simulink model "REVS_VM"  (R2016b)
settings: Solver=ode3  StartTime=REVS.sim_start_time_secs  StopTime=Inf  FixedStep=REVS.sim_step_time_secs  MaxStep=REVS.sim_step_time_secs  EnableMultiTasking=on
StopFcn:
  | postproc_datalog;
  | postproc_audit;
  | postproc_result;
model workspace (MATLAB code in the model file):
  other statements: REVS_setup_variants
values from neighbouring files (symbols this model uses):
  accessory = class_accessory_data    [class_test_data.m]
  battery = class_battery_data    [class_accessory_data.m]    (also in class_REVS_electric.m = class_REVS_battery)
  brake = struct(	'max_torque_Nm',[], 						'proportion_norm',1.0, 						'inertia_kgm2',0.0)    [class_REVS_drive_axle.m]
  engine = class_engine_data    [class_test_data.m]
  final_drive = struct(	'gear_ratio',[], 								'efficiency_norm',[], 								'inertia_kgm2',[] )    [class_REVS_drive_axle.m]
  gear = class_REVS_gearbox    [class_REVS_AT_transmission.m]
  tire = struct(	'radius_m',[], 						'rolling_resistance_coefficient',0, 						'vehicle_weight_norm',1.0,  						'wheel_slip_torque_Nm',[],  						'inertia_kgm2',0.0)    [class_REVS_drive_axle.m]
  torque_converter = class_REVS_torque_converter    [class_REVS_AT_transmission.m]
  transmission = class_transmission_data    [class_test_data.m]
  vehicle = class_vehicle_data    [class_test_data.m]
undefined symbols (not defined in the file or in its folder): alternator, ambient, controls, convert, DelayTimeSecs, drive_cycle, driver, electric, gear_strategy, InitialCondition, InitialValue, LoadSource, LookupStructure, MultiplyPosInputs, Normalize, NumPhases, REVS, SpeedSource, starter, tableshift, UpperSaturationLimit, Value, VerboseLevel, VerboseSignal
libraries: simulink x153
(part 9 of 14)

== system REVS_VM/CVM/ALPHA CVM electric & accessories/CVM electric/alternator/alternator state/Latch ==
  On : Inport  PortDimensions=1
  Off : Inport  Port=2  PortDimensions=1
  Combinatorial  Logic : CombinatorialLogic  TruthTable=[0;1;0;0;1;1;(tb==2);(tb>=2)]
  Memory2 : Memory  X0=InitialCondition
  Mux : Mux  Inputs=3
  State : Outport  PortDimensions=1
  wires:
  Off/1 -> Mux/2
  On/1 -> Mux/1
  Memory2/1 -> Mux/3
  Mux/1 -> Combinatorial  Logic/1
  Combinatorial  Logic/1 -> State/1, Memory2/1

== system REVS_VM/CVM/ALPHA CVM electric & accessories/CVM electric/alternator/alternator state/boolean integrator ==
  bool : Inport
  Constant : Constant  Value=Normalize
  Data Type Conversion2 : DataTypeConversion  OutDataTypeStr=double
  Integrator1 : Integrator  ExternalReset=falling  LimitOutput=on  UpperSaturationLimit=UpperSaturationLimit  LowerSaturationLimit=0
  Switch : Switch  Criteria=u2 > Threshold
  normalize : Gain  Gain=1/UpperSaturationLimit
  out : Outport
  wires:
  Switch/1 -> out/1
  normalize/1 -> Switch/1
  Integrator1/1 -> Switch/3, normalize/1
  Constant/1 -> Switch/2
  bool/1 -> Data Type Conversion2/1
  Data Type Conversion2/1 -> Integrator1/1, Integrator1/2

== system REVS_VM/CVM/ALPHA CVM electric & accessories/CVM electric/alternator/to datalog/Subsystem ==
  In1 : Inport
  Enable : EnablePort
  To Workspace : ToWorkspace  VariableName=datalog__alternator__regen_SOC_state  SampleTime=-1
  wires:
  In1/1 -> To Workspace/1

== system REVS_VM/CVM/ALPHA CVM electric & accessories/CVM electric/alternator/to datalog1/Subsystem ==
  In1 : Inport
  Enable : EnablePort
  To Workspace : ToWorkspace  VariableName=datalog__alternator__target_voltage  SampleTime=-1
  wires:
  In1/1 -> To Workspace/1

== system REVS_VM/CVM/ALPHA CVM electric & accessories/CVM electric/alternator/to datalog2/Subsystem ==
  In1 : Inport
  Enable : EnablePort
  To Workspace : ToWorkspace  VariableName=datalog__alternator__state  SampleTime=-1
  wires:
  In1/1 -> To Workspace/1

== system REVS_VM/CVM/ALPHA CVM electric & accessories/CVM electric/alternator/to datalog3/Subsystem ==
  In1 : Inport
  Enable : EnablePort
  To Workspace : ToWorkspace  VariableName=datalog__alternator__regen_state  SampleTime=-1
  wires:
  In1/1 -> To Workspace/1

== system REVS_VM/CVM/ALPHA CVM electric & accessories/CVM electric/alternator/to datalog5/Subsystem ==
  In1 : Inport
  Enable : EnablePort
  To Workspace : ToWorkspace  VariableName=datalog__alternator__upshift_sig  SampleTime=-1
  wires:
  In1/1 -> To Workspace/1

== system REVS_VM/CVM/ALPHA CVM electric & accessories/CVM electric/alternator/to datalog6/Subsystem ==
  In1 : Inport
  Enable : EnablePort
  To Workspace : ToWorkspace  VariableName=datalog__alternator__voltage_boost  SampleTime=-1
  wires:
  In1/1 -> To Workspace/1

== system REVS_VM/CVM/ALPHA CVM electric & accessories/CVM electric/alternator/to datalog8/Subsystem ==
  In1 : Inport
  Enable : EnablePort
  To Workspace : ToWorkspace  VariableName=datalog__alternator__PID_current_A  SampleTime=-1
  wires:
  In1/1 -> To Workspace/1

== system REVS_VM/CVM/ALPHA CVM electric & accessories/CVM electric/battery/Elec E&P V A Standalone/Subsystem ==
  volts_V : Inport
  curr_A : Inport  Port=2
  Enable : EnablePort  ZeroCross=off
  Elec Energy V A : Subsystem  TreatAsAtomicUnit=on
  amps_to_workspace : ToWorkspace  VariableName=audit__elec__battery_Amps  SampleTime=-1
  energy_to_workspace : ToWorkspace  VariableName=audit__elec__battery_kJ  SampleTime=-1
  neg_energy_to_workspace : ToWorkspace  VariableName=audit__elec__battery_neg_kJ  SampleTime=-1
  pos_energy_to_workspace : ToWorkspace  VariableName=audit__elec__battery_pos_kJ  SampleTime=-1
  power_to_workspace : ToWorkspace  VariableName=audit__elec__battery_kW  SampleTime=-1
  volts_to_workspace : ToWorkspace  VariableName=audit__elec__battery_Volts  SampleTime=-1
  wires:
  Elec Energy V A/1("total_kJ ") -> energy_to_workspace/1
  Elec Energy V A/4(pwr_kW) -> power_to_workspace/1
  Elec Energy V A/2("pos_kJ ") -> pos_energy_to_workspace/1
  Elec Energy V A/3(neg_kJ) -> neg_energy_to_workspace/1
  curr_A/1 -> amps_to_workspace/1, Elec Energy V A/2(curr_A)
  volts_V/1 -> volts_to_workspace/1, Elec Energy V A/1(volts_V)

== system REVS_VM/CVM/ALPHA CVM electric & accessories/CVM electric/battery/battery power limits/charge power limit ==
  bus : Inport
  Bus Selector : BusSelector  OutputSignals=gb.gb_cmd_gear,gb_spd_in_radps,ctrl.gb_line_press_bar
  Lookup : Lookup_n-D  NumberOfTableDimensions=10  BreakpointsForDimension1=LookupStructure.axis_1.breakpoints  BreakpointsForDimension2=LookupStructure.axis_2.breakpoints  BreakpointsForDimension3=LookupStructure.axis_3.breakpoints  BreakpointsForDimension4=LookupStructure.axis_4.breakpoints  BreakpointsForDimension5=LookupStructure.axis_5.breakpoints  BreakpointsForDimension6=LookupStructure.axis_6.breakpoints  BreakpointsForDimension7=LookupStructure.axis_7.breakpoints  BreakpointsForDimension8=LookupStructure.axis_8.breakpoints  BreakpointsForDimension9=LookupStructure.axis_9.breakpoints  BreakpointsForDimension10=LookupStructure.axis_10.breakpoints  IndexSearchMethod=Linear search  BeginIndexSearchUsingPreviousIndexResult=on  Table=LookupStructure.table  InternalRulePriority=Speed  RndMeth=Simplest  SupportTunableTableSize=on  MaximumIndicesForEachDimension=LookupStructure.table_size
  out : Outport
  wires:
  bus/1 -> Bus Selector/1
  Lookup/1 -> out/1

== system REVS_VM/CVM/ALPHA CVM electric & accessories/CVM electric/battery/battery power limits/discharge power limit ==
  bus : Inport
  Bus Selector : BusSelector  OutputSignals=gb.gb_cmd_gear,gb_spd_in_radps,ctrl.gb_line_press_bar
  Lookup : Lookup_n-D  NumberOfTableDimensions=10  BreakpointsForDimension1=LookupStructure.axis_1.breakpoints  BreakpointsForDimension2=LookupStructure.axis_2.breakpoints  BreakpointsForDimension3=LookupStructure.axis_3.breakpoints  BreakpointsForDimension4=LookupStructure.axis_4.breakpoints  BreakpointsForDimension5=LookupStructure.axis_5.breakpoints  BreakpointsForDimension6=LookupStructure.axis_6.breakpoints  BreakpointsForDimension7=LookupStructure.axis_7.breakpoints  BreakpointsForDimension8=LookupStructure.axis_8.breakpoints  BreakpointsForDimension9=LookupStructure.axis_9.breakpoints  BreakpointsForDimension10=LookupStructure.axis_10.breakpoints  IndexSearchMethod=Linear search  BeginIndexSearchUsingPreviousIndexResult=on  Table=LookupStructure.table  InternalRulePriority=Speed  RndMeth=Simplest  SupportTunableTableSize=on  MaximumIndicesForEachDimension=LookupStructure.table_size
  out : Outport
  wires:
  bus/1 -> Bus Selector/1
  Lookup/1 -> out/1

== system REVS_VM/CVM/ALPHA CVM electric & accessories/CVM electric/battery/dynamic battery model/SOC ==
  batt_curr_A : Inport
  batt_temp_degC : Inport  Port=2
  Bus Creator : BusCreator  Inputs=2
  Divide1 : Product  Inputs=*/
  Integrator : Integrator  InitialConditionSource=external  InitialCondition=battery.initial_soc_norm * battery.capacity_Coulombs  LimitOutput=on  UpperSaturationLimit=battery.capacity_Coulombs  LowerSaturationLimit=0
  Negative Gain1 : Gain  Gain=-1
  Product : Product
  Product1 : Product
  Switch : Switch  OutDataTypeStr=double
  capacity (Coulombs) : Constant  Value=battery.capacity_Coulombs
  charge efficiency dynamic : Subsystem
  initial SoC : Constant  Value=battery.initial_soc_norm
  to datalog with base name : Subsystem
  SoC_norm : Outport
  chg_eff_norm : Outport  Port=2
  pile_curr_A : Outport  Port=3
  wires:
  initial SoC/1 -> Product1/1
  Product1/1 -> Integrator/2
  Divide1/1 -> to datalog with base name/1(Var), Bus Creator/2, SoC_norm/1  "soc_norm"
  capacity (Coulombs)/1 -> Divide1/2, Product1/2
  Integrator/1 -> Divide1/1
  batt_temp_degC/1 -> Bus Creator/1  "temp_degC"
  batt_curr_A/1 -> Product/1, Switch/1, Switch/2
  Switch/1 -> Negative Gain1/1
  Product/1 -> Switch/3
  Negative Gain1/1 -> pile_curr_A/1, Integrator/1
  charge efficiency dynamic/1(out) -> chg_eff_norm/1, Product/2
  Bus Creator/1 -> charge efficiency dynamic/1(bus)

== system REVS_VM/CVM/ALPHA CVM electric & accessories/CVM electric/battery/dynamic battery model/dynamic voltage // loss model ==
  batt_curr_A : Inport
  SoC_norm : Inport  Port=2
  batt_temp_degC : Inport  Port=3
  chg_eff_norm : Inport  Port=4
  pile_curr_A : Inport  Port=5
  Add1 : Sum
  Add2 : Sum  Inputs=+-
  Bus Creator : BusCreator  Inputs=4
  Divide : Product  Inputs=*/
  Gain3 : Gain  Gain=battery.voltage_transient_cal_norm
  Gain4 : Gain  Gain=1/1000
  Gain5 : Gain  Gain=1/1000
  Integrator1 : Integrator  ZeroCross=off
  Integrator2 : Integrator  ZeroCross=off
  Integrator3 : Integrator  ZeroCross=off
  Product : Product
  Product1 : Product
  RC long term (LT) : Subsystem
  RC short term (ST) : Subsystem
  Rs : Subsystem
  Subtract1 : Sum  Inputs=+++
  battery energy change : Subsystem
  battery energy discharge gross : Subsystem
  battery loss : Subsystem
  battery loss1 : Subsystem
  charge loss : Subsystem
  model : Subsystem
  negative : Saturate  UpperLimit=0  LowerLimit=-Inf
  num parallels : Constant  Value=battery.num_parallel_cells
  open circuit (pile) voltage : Subsystem
  result integrator : Subsystem
  OCV_V : Outport
  batt_volts_V : Outport  Port=2
  dis_res_Ohm : Outport  Port=3
  chg_res_Ohm : Outport  Port=4
  loss_pwr_W : Outport  Port=5
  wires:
  Gain5/1 -> Integrator1/1, result integrator/1(in), negative/1
  negative/1 -> Integrator3/1
  Integrator3/1 -> battery energy discharge gross/1(Var)
  chg_eff_norm/1 -> charge loss/1(charge_eff_norm)
  Add1/1 -> loss_pwr_W/1, Integrator2/1
  Add2/1 -> Gain3/1
  RC long term (LT)/1(RC_LT_V) -> Subtract1/2
  batt_temp_degC/1 -> Bus Creator/3  "temp_degC"
  RC short term (ST)/1(RC_ST_V) -> Subtract1/1
  Rs/1(Rs_V) -> Subtract1/3
  SoC_norm/1 -> Bus Creator/1  "soc_norm"
  Rs/2(Rs_dis_Ohm) -> dis_res_Ohm/1
  Rs/3(Rs_chg_Ohm) -> chg_res_Ohm/1
  pile_curr_A/1 -> Product/2
  Product/1 -> Gain5/1
  Integrator1/1 -> battery energy change/1(Var)
  Subtract1/1 -> Add2/2, Product1/2
  open circuit (pile) voltage/1(OCV_V) -> battery loss1/1(Var), Product/1, charge loss/3(OCV_V), Add2/1, OCV_V/1
  Divide/1 -> Bus Creator/2  "cell_curr_A"
  num parallels/1 -> Divide/2
  batt_curr_A/1 -> Bus Creator/4, charge loss/2(pack_curr_A), Divide/1, Product1/1  "pack_curr_A"
  Integrator2/1 -> Gain4/1
  charge loss/1(chg_loss_pwr_W) -> Add1/2
  Product1/1 -> Add1/1
  Gain4/1 -> battery loss/1(Var)
  Bus Creator/1 -> Rs/1(bus_in), RC long term (LT)/1(bus_in), RC short term (ST)/1(bus_in), open circuit (pile) voltage/1(bus_in)
  Gain3/1 -> batt_volts_V/1

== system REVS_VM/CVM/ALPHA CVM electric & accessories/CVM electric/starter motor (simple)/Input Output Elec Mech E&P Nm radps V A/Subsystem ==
  volts_in_V : Inport
  curr_in_A : Inport  Port=2
  trq_out_Nm : Inport  Port=3
  spd_out_radps : Inport  Port=4
  iner_out_kgm2 : Inport  Port=5
  Enable : EnablePort
  Elec E&P V A : Subsystem
  Loss_KJ_to_workspace : ToWorkspace  VariableName=audit__mech__starter__loss_kJ  SampleTime=-1
  Mech E&P Nm radps : Subsystem
  Pos : Saturate  UpperLimit=Inf  LowerLimit=0  ZeroCross=off
  Pos2 : Saturate  UpperLimit=Inf  LowerLimit=0  ZeroCross=off
  Sum : Sum  Inputs=+-|
  Sum1 : Sum  Inputs=|-+
  Sum2 : Sum
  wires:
  Pos2/1 -> Sum2/1
  Pos/1 -> Sum2/2
  trq_out_Nm/1 -> Mech E&P Nm radps/1(" trq_Nm")
  spd_out_radps/1 -> Mech E&P Nm radps/2(spd_radps)
  volts_in_V/1 -> Elec E&P V A/1(volts_V)
  curr_in_A/1 -> Elec E&P V A/2(curr_A)
  iner_out_kgm2/1 -> Mech E&P Nm radps/3(iner_kgm2)
  Mech E&P Nm radps/1(pos_kJ) -> Sum/2
  Elec E&P V A/2(neg_kJ) -> Sum1/1
  Mech E&P Nm radps/2(neg_kJ) -> Sum1/2
  Sum/1 -> Pos/1
  Sum1/1 -> Pos2/1
  Sum2/1 -> Loss_KJ_to_workspace/1
  Elec E&P V A/1(pos_kJ) -> Sum/1

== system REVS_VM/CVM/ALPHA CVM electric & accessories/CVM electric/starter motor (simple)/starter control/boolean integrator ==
  bool : Inport
  Constant : Constant  Value=Normalize
  Data Type Conversion2 : DataTypeConversion  OutDataTypeStr=double
  Integrator1 : Integrator  ExternalReset=falling  LimitOutput=on  UpperSaturationLimit=UpperSaturationLimit  LowerSaturationLimit=0
  Switch : Switch  Criteria=u2 > Threshold
  normalize : Gain  Gain=1/UpperSaturationLimit
  out : Outport
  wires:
  Switch/1 -> out/1
  normalize/1 -> Switch/1
  Integrator1/1 -> Switch/3, normalize/1
  Constant/1 -> Switch/2
  bool/1 -> Data Type Conversion2/1
  Data Type Conversion2/1 -> Integrator1/1, Integrator1/2

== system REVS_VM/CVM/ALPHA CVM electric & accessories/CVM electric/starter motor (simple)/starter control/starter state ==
  On : Inport  PortDimensions=1
  Off : Inport  Port=2  PortDimensions=1
  Combinatorial  Logic : CombinatorialLogic  TruthTable=[0;1;0;0;1;1;(tb==2);(tb>=2)]
  Memory2 : Memory  X0=InitialCondition
  Mux : Mux  Inputs=3
  State : Outport  PortDimensions=1
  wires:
  Off/1 -> Mux/2
  On/1 -> Mux/1
  Memory2/1 -> Mux/3
  Mux/1 -> Combinatorial  Logic/1
  Combinatorial  Logic/1 -> State/1, Memory2/1

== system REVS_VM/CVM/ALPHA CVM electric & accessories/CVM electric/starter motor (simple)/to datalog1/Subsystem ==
  In1 : Inport
  Enable : EnablePort
  To Workspace : ToWorkspace  VariableName=datalog__electric__starter_PID_torque_Nm  SampleTime=-1
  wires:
  In1/1 -> To Workspace/1

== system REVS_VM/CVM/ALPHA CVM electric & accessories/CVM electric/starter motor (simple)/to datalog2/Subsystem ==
  In1 : Inport
  Enable : EnablePort
  To Workspace : ToWorkspace  VariableName=datalog__electric__starter_state  SampleTime=-1
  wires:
  In1/1 -> To Workspace/1

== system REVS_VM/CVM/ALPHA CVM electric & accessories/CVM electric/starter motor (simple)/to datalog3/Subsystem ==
  In1 : Inport
  Enable : EnablePort
  To Workspace : ToWorkspace  VariableName=datalog__electric__starter_desired_torque_Nm  SampleTime=-1
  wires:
  In1/1 -> To Workspace/1

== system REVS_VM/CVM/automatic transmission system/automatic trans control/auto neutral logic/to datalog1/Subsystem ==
  In1 : Inport
  Enable : EnablePort
  To Workspace : ToWorkspace  VariableName=datalog__transmission__auto_neutral_command_bool  SampleTime=-1
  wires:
  In1/1 -> To Workspace/1

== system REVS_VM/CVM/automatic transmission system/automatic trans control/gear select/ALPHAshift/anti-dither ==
  raw : Inport
  Abs : Abs
  Memory : Memory
  Rounding Function : Rounding  Operator=round
  Sum : Sum  Inputs=|+-
  Switch : Switch  Criteria=u2 > Threshold  Threshold=.66
  low pass filter : TransferFcn  Denominator=[0.02 1]
  to datalog17 : Subsystem
  to datalog18 : Subsystem
  out : Outport
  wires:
  raw/1 -> to datalog18/1(Var), low pass filter/1
  low pass filter/1 -> Rounding Function/1, Sum/1, to datalog17/1(Var)
  Rounding Function/1 -> Switch/1
  Switch/1 -> out/1, Memory/1
  Sum/1 -> Abs/1
  Memory/1 -> Sum/2, Switch/3
  Abs/1 -> Switch/2

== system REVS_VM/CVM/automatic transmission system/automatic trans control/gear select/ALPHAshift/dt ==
  Clock : Clock
  Memory1 : Memory
  Sum : Sum  Inputs=|-+
  dt : Outport
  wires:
  Clock/1 -> Sum/2, Memory1/1
  Memory1/1 -> Sum/1
  Sum/1 -> dt/1

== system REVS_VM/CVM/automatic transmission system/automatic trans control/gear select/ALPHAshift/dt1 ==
  Clock : Clock
  Memory1 : Memory
  Sum : Sum  Inputs=|-+
  dt : Outport
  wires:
  Clock/1 -> Sum/2, Memory1/1
  Memory1/1 -> Sum/1
  Sum/1 -> dt/1

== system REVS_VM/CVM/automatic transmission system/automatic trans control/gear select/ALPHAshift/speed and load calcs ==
  eng_load_Nm : Inport
  trans_spd_in_radps : Inport  Port=2
  trans_spd_out_radps : Inport  Port=3
  eng_spd_radps : Inport  Port=4
  trans_gear_ratios : Inport  Port=5
  Logical Operator : Logic  Operator=NOT  AllPortsSameDT=off  OutDataTypeStr=boolean
  MinMax : MinMax  Inputs=2  ZeroCross=off
  MinMax1 : MinMax  Function=max  ZeroCross=off
  MinMax2 : MinMax  Function=max  Inputs=2  ZeroCross=off
  Product1 : Product  Inputs=***/
  Product2 : Product  Inputs=***
  Product3 : Product  Inputs=*/
  Product4 : Product  Inputs=***/
  Product5 : Product  Inputs=**
  Sum : Sum  Inputs=|++
  cost map : Lookup_n-D  BreakpointsForDimension1=gear_strategy.cost_map_torque_Nm  BreakpointsForDimension2=gear_strategy.cost_map_speed_radps  IndexSearchMethod=Linear search  BeginIndexSearchUsingPreviousIndexResult=on  Table=gear_strategy.cost_map  ExtrapMethod=Clip  UseLastTableValue=on  RndMeth=Simplest
  eps1 : Saturate  UpperLimit=Inf  LowerLimit=eps
  eps2 : Saturate  UpperLimit=Inf  LowerLimit=eps  ZeroCross=off
  eps3 : Saturate  UpperLimit=Inf  LowerLimit=eps
  max input torque : Lookup_n-D  NumberOfTableDimensions=1  BreakpointsForDimension1=gear_strategy.max_input_torque_speeds_radps  IndexSearchMethod=Linear search  BeginIndexSearchUsingPreviousIndexResult=on  Table=gear_strategy.max_input_torque_curve_Nm  ExtrapMethod=Clip  UseLastTableValue=on  RndMeth=Simplest
  non-neutral gears vector : simulink/Logic and Bit Operations/Compare To Zero  relop=~=  OutDataTypeStr=boolean
  non-neutral gears vector1 : simulink/Logic and Bit Operations/Compare To Zero  relop=~=  OutDataTypeStr=boolean
  speed mask : Constant  Value=gear_strategy.use_engine_speed_mask
  gear_trq_Nm : Outport
  gear_spd_radps : Outport  Port=2
  gear_cost : Outport  Port=3
  gear_avail_trq_Nm : Outport  Port=4
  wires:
  Product4/1 -> Sum/2  "engine_speeds"
  Product2/1 -> Sum/1  "speeds"
  eps3/1 -> Product4/4
  eng_spd_radps/1 -> Product1/3, MinMax2/2
  eng_load_Nm/1 -> Product1/1
  eps1/1 -> Product1/4
  non-neutral gears vector/1 -> Product1/2
  trans_gear_ratios/1 -> MinMax1/1, non-neutral gears vector/1, Product2/2, Product4/3, non-neutral gears vector1/1
  Sum/1 -> max input torque/1, cost map/2, eps1/1, gear_spd_radps/1  "speeds"
  Product1/1 -> cost map/1, gear_trq_Nm/1  "engine_loads"
  eps2/1 -> Product3/2
  Product3/1 -> MinMax/2
  MinMax/1 -> eps3/1
  MinMax1/1 -> MinMax/1
  trans_spd_in_radps/1 -> MinMax2/1, Product3/1
  trans_spd_out_radps/1 -> eps2/1, Product2/1
  max input torque/1 -> Product5/1
  Product5/1 -> gear_avail_trq_Nm/1
  non-neutral gears vector1/1 -> Product5/2
  cost map/1 -> gear_cost/1
  Logical Operator/1 -> Product2/3
  speed mask/1 -> Logical Operator/1, Product4/1
  MinMax2/1 -> Product4/2

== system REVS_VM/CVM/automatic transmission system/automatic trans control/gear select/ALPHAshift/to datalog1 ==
  Var : Inport
  Constant : Constant  Value=VerboseSignal
  Constant1 : Constant  Value=VerboseLevel
  Relational Operator : RelationalOperator  OutDataTypeStr=boolean  ZeroCross=off
  Subsystem : Subsystem
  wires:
  Constant1/1 -> Relational Operator/2
  Constant/1 -> Relational Operator/1
  Relational Operator/1 -> Subsystem/Enable
  Var/1 -> Subsystem/1(In1)

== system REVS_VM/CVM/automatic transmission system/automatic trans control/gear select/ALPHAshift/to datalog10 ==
  Var : Inport
  Constant : Constant  Value=VerboseSignal
  Constant1 : Constant  Value=VerboseLevel
  Relational Operator : RelationalOperator  OutDataTypeStr=boolean  ZeroCross=off
  Subsystem : Subsystem
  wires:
  Constant1/1 -> Relational Operator/2
  Constant/1 -> Relational Operator/1
  Relational Operator/1 -> Subsystem/Enable
  Var/1 -> Subsystem/1(In1)

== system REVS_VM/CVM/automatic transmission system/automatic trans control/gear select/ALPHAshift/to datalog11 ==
  Var : Inport
  Constant : Constant  Value=VerboseSignal
  Constant1 : Constant  Value=VerboseLevel
  Relational Operator : RelationalOperator  OutDataTypeStr=boolean  ZeroCross=off
  Subsystem : Subsystem
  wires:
  Constant1/1 -> Relational Operator/2
  Constant/1 -> Relational Operator/1
  Relational Operator/1 -> Subsystem/Enable
  Var/1 -> Subsystem/1(In1)

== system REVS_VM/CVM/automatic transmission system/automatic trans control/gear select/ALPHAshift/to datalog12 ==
  Var : Inport
  Constant : Constant  Value=VerboseSignal
  Constant1 : Constant  Value=VerboseLevel
  Relational Operator : RelationalOperator  OutDataTypeStr=boolean  ZeroCross=off
  Subsystem : Subsystem
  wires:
  Constant1/1 -> Relational Operator/2
  Constant/1 -> Relational Operator/1
  Relational Operator/1 -> Subsystem/Enable
  Var/1 -> Subsystem/1(In1)

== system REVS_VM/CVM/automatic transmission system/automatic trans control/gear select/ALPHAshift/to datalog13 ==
  Var : Inport
  Constant : Constant  Value=VerboseSignal
  Constant1 : Constant  Value=VerboseLevel
  Relational Operator : RelationalOperator  OutDataTypeStr=boolean  ZeroCross=off
  Subsystem : Subsystem
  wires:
  Constant1/1 -> Relational Operator/2
  Constant/1 -> Relational Operator/1
  Relational Operator/1 -> Subsystem/Enable
  Var/1 -> Subsystem/1(In1)

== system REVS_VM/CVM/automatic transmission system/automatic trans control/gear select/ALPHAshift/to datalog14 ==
  Var : Inport
  Constant : Constant  Value=VerboseSignal
  Constant1 : Constant  Value=VerboseLevel
  Relational Operator : RelationalOperator  OutDataTypeStr=boolean  ZeroCross=off
  Subsystem : Subsystem
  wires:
  Constant1/1 -> Relational Operator/2
  Constant/1 -> Relational Operator/1
  Relational Operator/1 -> Subsystem/Enable
  Var/1 -> Subsystem/1(In1)

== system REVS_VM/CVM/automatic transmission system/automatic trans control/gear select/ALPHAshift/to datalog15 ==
  Var : Inport
  Constant : Constant  Value=VerboseSignal
  Constant1 : Constant  Value=VerboseLevel
  Relational Operator : RelationalOperator  OutDataTypeStr=boolean  ZeroCross=off
  Subsystem : Subsystem
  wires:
  Constant1/1 -> Relational Operator/2
  Constant/1 -> Relational Operator/1
  Relational Operator/1 -> Subsystem/Enable
  Var/1 -> Subsystem/1(In1)

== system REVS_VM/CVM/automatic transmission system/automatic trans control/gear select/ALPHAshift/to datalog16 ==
  Var : Inport
  Constant : Constant  Value=VerboseSignal
  Constant1 : Constant  Value=VerboseLevel
  Relational Operator : RelationalOperator  OutDataTypeStr=boolean  ZeroCross=off
  Subsystem : Subsystem
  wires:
  Constant1/1 -> Relational Operator/2
  Constant/1 -> Relational Operator/1
  Relational Operator/1 -> Subsystem/Enable
  Var/1 -> Subsystem/1(In1)

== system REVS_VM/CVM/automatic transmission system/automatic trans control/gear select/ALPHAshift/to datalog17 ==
  Var : Inport
  Constant : Constant  Value=VerboseSignal
  Constant1 : Constant  Value=VerboseLevel
  Relational Operator : RelationalOperator  OutDataTypeStr=boolean  ZeroCross=off
  Subsystem : Subsystem
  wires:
  Constant1/1 -> Relational Operator/2
  Constant/1 -> Relational Operator/1
  Relational Operator/1 -> Subsystem/Enable
  Var/1 -> Subsystem/1(In1)

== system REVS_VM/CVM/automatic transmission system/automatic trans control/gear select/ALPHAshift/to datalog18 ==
  Var : Inport
  Constant : Constant  Value=VerboseSignal
  Constant1 : Constant  Value=VerboseLevel
  Relational Operator : RelationalOperator  OutDataTypeStr=boolean  ZeroCross=off
  Subsystem : Subsystem
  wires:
  Constant1/1 -> Relational Operator/2
  Constant/1 -> Relational Operator/1
  Relational Operator/1 -> Subsystem/Enable
  Var/1 -> Subsystem/1(In1)

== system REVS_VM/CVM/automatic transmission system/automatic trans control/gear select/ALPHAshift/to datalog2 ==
  Var : Inport
  Constant : Constant  Value=VerboseSignal
  Constant1 : Constant  Value=VerboseLevel
  Relational Operator : RelationalOperator  OutDataTypeStr=boolean  ZeroCross=off
  Subsystem : Subsystem
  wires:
  Constant1/1 -> Relational Operator/2
  Constant/1 -> Relational Operator/1
  Relational Operator/1 -> Subsystem/Enable
  Var/1 -> Subsystem/1(In1)

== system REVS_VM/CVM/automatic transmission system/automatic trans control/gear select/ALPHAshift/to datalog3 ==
  Var : Inport
  Constant : Constant  Value=VerboseSignal
  Constant1 : Constant  Value=VerboseLevel
  Relational Operator : RelationalOperator  OutDataTypeStr=boolean  ZeroCross=off
  Subsystem : Subsystem
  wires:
  Constant1/1 -> Relational Operator/2
  Constant/1 -> Relational Operator/1
  Relational Operator/1 -> Subsystem/Enable
  Var/1 -> Subsystem/1(In1)

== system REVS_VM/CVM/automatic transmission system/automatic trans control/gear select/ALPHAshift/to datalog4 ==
  Var : Inport
  Constant : Constant  Value=VerboseSignal
  Constant1 : Constant  Value=VerboseLevel
  Relational Operator : RelationalOperator  OutDataTypeStr=boolean  ZeroCross=off
  Subsystem : Subsystem
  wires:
  Constant1/1 -> Relational Operator/2
  Constant/1 -> Relational Operator/1
  Relational Operator/1 -> Subsystem/Enable
  Var/1 -> Subsystem/1(In1)

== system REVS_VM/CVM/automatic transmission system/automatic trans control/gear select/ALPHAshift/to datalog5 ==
  Var : Inport
  Constant : Constant  Value=VerboseSignal
  Constant1 : Constant  Value=VerboseLevel
  Relational Operator : RelationalOperator  OutDataTypeStr=boolean  ZeroCross=off
  Subsystem : Subsystem
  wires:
  Constant1/1 -> Relational Operator/2
  Constant/1 -> Relational Operator/1
  Relational Operator/1 -> Subsystem/Enable
  Var/1 -> Subsystem/1(In1)

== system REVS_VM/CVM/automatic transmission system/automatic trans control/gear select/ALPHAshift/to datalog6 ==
  Var : Inport
  Constant : Constant  Value=VerboseSignal
  Constant1 : Constant  Value=VerboseLevel
  Relational Operator : RelationalOperator  OutDataTypeStr=boolean  ZeroCross=off
  Subsystem : Subsystem
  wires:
  Constant1/1 -> Relational Operator/2
  Constant/1 -> Relational Operator/1
  Relational Operator/1 -> Subsystem/Enable
  Var/1 -> Subsystem/1(In1)

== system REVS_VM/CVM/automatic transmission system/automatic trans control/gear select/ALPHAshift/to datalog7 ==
  Var : Inport
  Constant : Constant  Value=VerboseSignal
  Constant1 : Constant  Value=VerboseLevel
  Relational Operator : RelationalOperator  OutDataTypeStr=boolean  ZeroCross=off
  Subsystem : Subsystem
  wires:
  Constant1/1 -> Relational Operator/2
  Constant/1 -> Relational Operator/1
  Relational Operator/1 -> Subsystem/Enable
  Var/1 -> Subsystem/1(In1)

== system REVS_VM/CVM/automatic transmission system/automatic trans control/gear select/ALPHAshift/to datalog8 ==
  Var : Inport
  Constant : Constant  Value=VerboseSignal
  Constant1 : Constant  Value=VerboseLevel
  Relational Operator : RelationalOperator  OutDataTypeStr=boolean  ZeroCross=off
  Subsystem : Subsystem
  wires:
  Constant1/1 -> Relational Operator/2
  Constant/1 -> Relational Operator/1
  Relational Operator/1 -> Subsystem/Enable
  Var/1 -> Subsystem/1(In1)

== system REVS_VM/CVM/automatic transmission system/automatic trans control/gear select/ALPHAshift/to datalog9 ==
  Var : Inport
  Constant : Constant  Value=VerboseSignal
  Constant1 : Constant  Value=VerboseLevel
  Relational Operator : RelationalOperator  OutDataTypeStr=boolean  ZeroCross=off
  Subsystem : Subsystem
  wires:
  Constant1/1 -> Relational Operator/2
  Constant/1 -> Relational Operator/1
  Relational Operator/1 -> Subsystem/Enable
  Var/1 -> Subsystem/1(In1)

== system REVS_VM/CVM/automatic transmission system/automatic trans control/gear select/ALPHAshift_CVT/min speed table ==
  bus : Inport
  Bus Selector : BusSelector  OutputSignals=gb.gb_cmd_gear,gb_spd_in_radps,ctrl.gb_line_press_bar
  Lookup : Lookup_n-D  NumberOfTableDimensions=10  BreakpointsForDimension1=LookupStructure.axis_1.breakpoints  BreakpointsForDimension2=LookupStructure.axis_2.breakpoints  BreakpointsForDimension3=LookupStructure.axis_3.breakpoints  BreakpointsForDimension4=LookupStructure.axis_4.breakpoints  BreakpointsForDimension5=LookupStructure.axis_5.breakpoints  BreakpointsForDimension6=LookupStructure.axis_6.breakpoints  BreakpointsForDimension7=LookupStructure.axis_7.breakpoints  BreakpointsForDimension8=LookupStructure.axis_8.breakpoints  BreakpointsForDimension9=LookupStructure.axis_9.breakpoints  BreakpointsForDimension10=LookupStructure.axis_10.breakpoints  IndexSearchMethod=Linear search  BeginIndexSearchUsingPreviousIndexResult=on  Table=LookupStructure.table  DiagnosticForOutOfRangeInput=Warning  InternalRulePriority=Speed  RndMeth=Simplest  SupportTunableTableSize=on  MaximumIndicesForEachDimension=LookupStructure.table_size
  out : Outport
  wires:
  bus/1 -> Bus Selector/1
  Lookup/1 -> out/1

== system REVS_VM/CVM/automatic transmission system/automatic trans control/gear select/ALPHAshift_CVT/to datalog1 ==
  Var : Inport
  Constant : Constant  Value=VerboseSignal
  Constant1 : Constant  Value=VerboseLevel
  Relational Operator : RelationalOperator  OutDataTypeStr=boolean  ZeroCross=off
  Subsystem : Subsystem
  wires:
  Constant1/1 -> Relational Operator/2
  Constant/1 -> Relational Operator/1
  Relational Operator/1 -> Subsystem/Enable
  Var/1 -> Subsystem/1(In1)

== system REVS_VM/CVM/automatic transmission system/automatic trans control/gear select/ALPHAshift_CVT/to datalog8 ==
  Var : Inport
  Constant : Constant  Value=VerboseSignal
  Constant1 : Constant  Value=VerboseLevel
  Relational Operator : RelationalOperator  OutDataTypeStr=boolean  ZeroCross=off
  Subsystem : Subsystem
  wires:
  Constant1/1 -> Relational Operator/2
  Constant/1 -> Relational Operator/1
  Relational Operator/1 -> Subsystem/Enable
  Var/1 -> Subsystem/1(In1)

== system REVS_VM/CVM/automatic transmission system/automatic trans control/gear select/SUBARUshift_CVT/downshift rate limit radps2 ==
  bus : Inport
  Bus Selector : BusSelector  OutputSignals=gb.gb_cmd_gear,gb_spd_in_radps,ctrl.gb_line_press_bar
  Lookup : Lookup_n-D  NumberOfTableDimensions=10  BreakpointsForDimension1=LookupStructure.axis_1.breakpoints  BreakpointsForDimension2=LookupStructure.axis_2.breakpoints  BreakpointsForDimension3=LookupStructure.axis_3.breakpoints  BreakpointsForDimension4=LookupStructure.axis_4.breakpoints  BreakpointsForDimension5=LookupStructure.axis_5.breakpoints  BreakpointsForDimension6=LookupStructure.axis_6.breakpoints  BreakpointsForDimension7=LookupStructure.axis_7.breakpoints  BreakpointsForDimension8=LookupStructure.axis_8.breakpoints  BreakpointsForDimension9=LookupStructure.axis_9.breakpoints  BreakpointsForDimension10=LookupStructure.axis_10.breakpoints  IndexSearchMethod=Linear search  BeginIndexSearchUsingPreviousIndexResult=on  Table=LookupStructure.table  InternalRulePriority=Speed  RndMeth=Simplest  SupportTunableTableSize=on  MaximumIndicesForEachDimension=LookupStructure.table_size
  out : Outport
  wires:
  bus/1 -> Bus Selector/1
  Lookup/1 -> out/1

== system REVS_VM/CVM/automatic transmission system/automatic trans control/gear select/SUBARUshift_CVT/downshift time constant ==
  bus : Inport
  Bus Selector : BusSelector  OutputSignals=gb.gb_cmd_gear,gb_spd_in_radps,ctrl.gb_line_press_bar
  Lookup : Lookup_n-D  NumberOfTableDimensions=10  BreakpointsForDimension1=LookupStructure.axis_1.breakpoints  BreakpointsForDimension2=LookupStructure.axis_2.breakpoints  BreakpointsForDimension3=LookupStructure.axis_3.breakpoints  BreakpointsForDimension4=LookupStructure.axis_4.breakpoints  BreakpointsForDimension5=LookupStructure.axis_5.breakpoints  BreakpointsForDimension6=LookupStructure.axis_6.breakpoints  BreakpointsForDimension7=LookupStructure.axis_7.breakpoints  BreakpointsForDimension8=LookupStructure.axis_8.breakpoints  BreakpointsForDimension9=LookupStructure.axis_9.breakpoints  BreakpointsForDimension10=LookupStructure.axis_10.breakpoints  IndexSearchMethod=Linear search  BeginIndexSearchUsingPreviousIndexResult=on  Table=LookupStructure.table  InternalRulePriority=Speed  RndMeth=Simplest  SupportTunableTableSize=on  MaximumIndicesForEachDimension=LookupStructure.table_size
  out : Outport
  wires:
  bus/1 -> Bus Selector/1
  Lookup/1 -> out/1

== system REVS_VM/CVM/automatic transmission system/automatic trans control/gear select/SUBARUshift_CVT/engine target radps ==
  bus : Inport
  Bus Selector : BusSelector  OutputSignals=gb.gb_cmd_gear,gb_spd_in_radps,ctrl.gb_line_press_bar
  Lookup : Lookup_n-D  NumberOfTableDimensions=10  BreakpointsForDimension1=LookupStructure.axis_1.breakpoints  BreakpointsForDimension2=LookupStructure.axis_2.breakpoints  BreakpointsForDimension3=LookupStructure.axis_3.breakpoints  BreakpointsForDimension4=LookupStructure.axis_4.breakpoints  BreakpointsForDimension5=LookupStructure.axis_5.breakpoints  BreakpointsForDimension6=LookupStructure.axis_6.breakpoints  BreakpointsForDimension7=LookupStructure.axis_7.breakpoints  BreakpointsForDimension8=LookupStructure.axis_8.breakpoints  BreakpointsForDimension9=LookupStructure.axis_9.breakpoints  BreakpointsForDimension10=LookupStructure.axis_10.breakpoints  IndexSearchMethod=Linear search  BeginIndexSearchUsingPreviousIndexResult=on  Table=LookupStructure.table  InternalRulePriority=Speed  RndMeth=Simplest  SupportTunableTableSize=on  MaximumIndicesForEachDimension=LookupStructure.table_size
  out : Outport
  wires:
  bus/1 -> Bus Selector/1
  Lookup/1 -> out/1

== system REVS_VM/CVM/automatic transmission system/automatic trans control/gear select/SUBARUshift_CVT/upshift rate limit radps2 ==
  bus : Inport
  Bus Selector : BusSelector  OutputSignals=gb.gb_cmd_gear,gb_spd_in_radps,ctrl.gb_line_press_bar
  Lookup : Lookup_n-D  NumberOfTableDimensions=10  BreakpointsForDimension1=LookupStructure.axis_1.breakpoints  BreakpointsForDimension2=LookupStructure.axis_2.breakpoints  BreakpointsForDimension3=LookupStructure.axis_3.breakpoints  BreakpointsForDimension4=LookupStructure.axis_4.breakpoints  BreakpointsForDimension5=LookupStructure.axis_5.breakpoints  BreakpointsForDimension6=LookupStructure.axis_6.breakpoints  BreakpointsForDimension7=LookupStructure.axis_7.breakpoints  BreakpointsForDimension8=LookupStructure.axis_8.breakpoints  BreakpointsForDimension9=LookupStructure.axis_9.breakpoints  BreakpointsForDimension10=LookupStructure.axis_10.breakpoints  IndexSearchMethod=Linear search  BeginIndexSearchUsingPreviousIndexResult=on  Table=LookupStructure.table  InternalRulePriority=Speed  RndMeth=Simplest  SupportTunableTableSize=on  MaximumIndicesForEachDimension=LookupStructure.table_size
  out : Outport
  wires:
  bus/1 -> Bus Selector/1
  Lookup/1 -> out/1

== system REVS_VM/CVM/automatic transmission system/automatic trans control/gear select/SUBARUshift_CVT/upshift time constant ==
  bus : Inport
  Bus Selector : BusSelector  OutputSignals=gb.gb_cmd_gear,gb_spd_in_radps,ctrl.gb_line_press_bar
  Lookup : Lookup_n-D  NumberOfTableDimensions=10  BreakpointsForDimension1=LookupStructure.axis_1.breakpoints  BreakpointsForDimension2=LookupStructure.axis_2.breakpoints  BreakpointsForDimension3=LookupStructure.axis_3.breakpoints  BreakpointsForDimension4=LookupStructure.axis_4.breakpoints  BreakpointsForDimension5=LookupStructure.axis_5.breakpoints  BreakpointsForDimension6=LookupStructure.axis_6.breakpoints  BreakpointsForDimension7=LookupStructure.axis_7.breakpoints  BreakpointsForDimension8=LookupStructure.axis_8.breakpoints  BreakpointsForDimension9=LookupStructure.axis_9.breakpoints  BreakpointsForDimension10=LookupStructure.axis_10.breakpoints  IndexSearchMethod=Linear search  BeginIndexSearchUsingPreviousIndexResult=on  Table=LookupStructure.table  InternalRulePriority=Speed  RndMeth=Simplest  SupportTunableTableSize=on  MaximumIndicesForEachDimension=LookupStructure.table_size
  out : Outport
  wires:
  bus/1 -> Bus Selector/1
  Lookup/1 -> out/1

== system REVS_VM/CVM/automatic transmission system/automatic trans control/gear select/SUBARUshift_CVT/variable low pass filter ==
  in : Inport
  time const : Inport  Port=2
  Add1 : Sum  Inputs=+-
  Add2 : Sum
  Constant1 : Constant  Value=-1
  Math Function : Math
  Memory : Memory  X0=max(transmission.gear.ratio)
  Product2 : Product
  Product3 : Product  Inputs=**/
  dt : Subsystem
  out : Outport
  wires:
  time const/1 -> Product3/3
  in/1 -> Add1/2, Add2/2
  Product3/1 -> Math Function/1
  Constant1/1 -> Product3/1
  Math Function/1 -> Product2/2
  Product2/1 -> Add2/1
  Add1/1 -> Product2/1
  Memory/1 -> Add1/1
  Add2/1 -> Memory/1, out/1
  dt/1(dt) -> Product3/2

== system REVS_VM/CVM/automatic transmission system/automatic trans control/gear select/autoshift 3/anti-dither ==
  raw : Inport
  Abs : Abs
  Memory : Memory
  Rounding Function : Rounding  Operator=round
  Sum : Sum  Inputs=|+-
  Switch : Switch  Criteria=u2 > Threshold  Threshold=.66
  low pass filter : TransferFcn  Denominator=[0.02 1]
  to datalog17 : Subsystem
  to datalog18 : Subsystem
  out : Outport
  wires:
  Abs/1 -> Switch/2
  Memory/1 -> Switch/3, Sum/2
  Sum/1 -> Abs/1
  Switch/1 -> Memory/1, out/1
  Rounding Function/1 -> Switch/1
  low pass filter/1 -> to datalog17/1(Var), Sum/1, Rounding Function/1
  raw/1 -> low pass filter/1, to datalog18/1(Var)

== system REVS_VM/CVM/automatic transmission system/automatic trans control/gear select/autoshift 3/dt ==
  Clock : Clock
  Memory1 : Memory
  Sum : Sum  Inputs=|-+
  dt : Outport
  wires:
  Clock/1 -> Sum/2, Memory1/1
  Memory1/1 -> Sum/1
  Sum/1 -> dt/1

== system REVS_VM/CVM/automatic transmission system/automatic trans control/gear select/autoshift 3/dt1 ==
  Clock : Clock
  Memory1 : Memory
  Sum : Sum  Inputs=|-+
  dt : Outport
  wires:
  Clock/1 -> Sum/2, Memory1/1
  Memory1/1 -> Sum/1
  Sum/1 -> dt/1

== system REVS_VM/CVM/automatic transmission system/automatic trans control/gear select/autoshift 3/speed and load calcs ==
  eng_load_Nm : Inport
  trans_spd_in_radps : Inport  Port=2
  trans_spd_out_radps : Inport  Port=3
  eng_spd_radps : Inport  Port=4
  trans_gear_ratios : Inport  Port=5
  Logical Operator : Logic  Operator=NOT  AllPortsSameDT=off  OutDataTypeStr=boolean
  MinMax : MinMax  Inputs=2  ZeroCross=off
  MinMax1 : MinMax  Function=max  ZeroCross=off
  MinMax2 : MinMax  Function=max  Inputs=2  ZeroCross=off
  Product1 : Product  Inputs=***/
  Product2 : Product  Inputs=***
  Product3 : Product  Inputs=*/
  Product4 : Product  Inputs=***/
  Product5 : Product  Inputs=**
  Sum : Sum  Inputs=|++
  cost map : Lookup_n-D  BreakpointsForDimension1=gear_strategy.cost_map_torque_Nm  BreakpointsForDimension2=gear_strategy.cost_map_speed_radps  IndexSearchMethod=Linear search  BeginIndexSearchUsingPreviousIndexResult=on  Table=gear_strategy.cost_map  ExtrapMethod=Clip  UseLastTableValue=on  RndMeth=Simplest
  eps1 : Saturate  UpperLimit=Inf  LowerLimit=eps
  eps2 : Saturate  UpperLimit=Inf  LowerLimit=eps  ZeroCross=off
  eps3 : Saturate  UpperLimit=Inf  LowerLimit=eps
  max input torque : Lookup_n-D  NumberOfTableDimensions=1  BreakpointsForDimension1=gear_strategy.max_input_torque_speeds_radps  IndexSearchMethod=Linear search  BeginIndexSearchUsingPreviousIndexResult=on  Table=gear_strategy.max_input_torque_curve_Nm  ExtrapMethod=Clip  UseLastTableValue=on  RndMeth=Simplest
  non-neutral gears vector : simulink/Logic and Bit Operations/Compare To Zero  relop=~=  OutDataTypeStr=boolean
  non-neutral gears vector1 : simulink/Logic and Bit Operations/Compare To Zero  relop=~=  OutDataTypeStr=boolean
  speed mask : Constant  Value=gear_strategy.use_engine_speed_mask
  gear_trq_Nm : Outport
  gear_spd_radps : Outport  Port=2
  gear_cost : Outport  Port=3
  gear_avail_trq_Nm : Outport  Port=4
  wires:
  MinMax2/1 -> Product4/2
  speed mask/1 -> Product4/1, Logical Operator/1
  Logical Operator/1 -> Product2/3
  cost map/1 -> gear_cost/1
  non-neutral gears vector1/1 -> Product5/2
  Product5/1 -> gear_avail_trq_Nm/1
  max input torque/1 -> Product5/1
  trans_spd_out_radps/1 -> Product2/1, eps2/1
  trans_spd_in_radps/1 -> Product3/1, MinMax2/1
  MinMax1/1 -> MinMax/1
  MinMax/1 -> eps3/1
  Product3/1 -> MinMax/2
  eps2/1 -> Product3/2
  Product1/1 -> gear_trq_Nm/1, cost map/1  "engine_loads"
  Sum/1 -> gear_spd_radps/1, eps1/1, cost map/2, max input torque/1  "speeds"
  trans_gear_ratios/1 -> non-neutral gears vector1/1, Product4/3, Product2/2, non-neutral gears vector/1, MinMax1/1
  non-neutral gears vector/1 -> Product1/2
  eps1/1 -> Product1/4
  eng_load_Nm/1 -> Product1/1
  eng_spd_radps/1 -> MinMax2/2, Product1/3
  eps3/1 -> Product4/4
  Product2/1 -> Sum/1  "speeds"
  Product4/1 -> Sum/2  "engine_speeds"

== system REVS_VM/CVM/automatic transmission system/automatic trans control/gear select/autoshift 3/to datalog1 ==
  Var : Inport
  Constant : Constant  Value=VerboseSignal
  Constant1 : Constant  Value=VerboseLevel
  Relational Operator : RelationalOperator  OutDataTypeStr=boolean  ZeroCross=off
  Subsystem : Subsystem
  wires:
  Constant1/1 -> Relational Operator/2
  Constant/1 -> Relational Operator/1
  Relational Operator/1 -> Subsystem/Enable
  Var/1 -> Subsystem/1(In1)

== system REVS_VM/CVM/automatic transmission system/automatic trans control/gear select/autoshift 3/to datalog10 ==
  Var : Inport
  Constant : Constant  Value=VerboseSignal
  Constant1 : Constant  Value=VerboseLevel
  Relational Operator : RelationalOperator  OutDataTypeStr=boolean  ZeroCross=off
  Subsystem : Subsystem
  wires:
  Constant1/1 -> Relational Operator/2
  Constant/1 -> Relational Operator/1
  Relational Operator/1 -> Subsystem/Enable
  Var/1 -> Subsystem/1(In1)

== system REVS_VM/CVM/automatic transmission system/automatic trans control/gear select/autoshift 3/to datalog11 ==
  Var : Inport
  Constant : Constant  Value=VerboseSignal
  Constant1 : Constant  Value=VerboseLevel
  Relational Operator : RelationalOperator  OutDataTypeStr=boolean  ZeroCross=off
  Subsystem : Subsystem
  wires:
  Constant1/1 -> Relational Operator/2
  Constant/1 -> Relational Operator/1
  Relational Operator/1 -> Subsystem/Enable
  Var/1 -> Subsystem/1(In1)

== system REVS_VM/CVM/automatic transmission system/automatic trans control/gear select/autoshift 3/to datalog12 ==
  Var : Inport
  Constant : Constant  Value=VerboseSignal
  Constant1 : Constant  Value=VerboseLevel
  Relational Operator : RelationalOperator  OutDataTypeStr=boolean  ZeroCross=off
  Subsystem : Subsystem
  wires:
  Constant1/1 -> Relational Operator/2
  Constant/1 -> Relational Operator/1
  Relational Operator/1 -> Subsystem/Enable
  Var/1 -> Subsystem/1(In1)

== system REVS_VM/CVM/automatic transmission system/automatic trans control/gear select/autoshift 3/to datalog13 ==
  Var : Inport
  Constant : Constant  Value=VerboseSignal
  Constant1 : Constant  Value=VerboseLevel
  Relational Operator : RelationalOperator  OutDataTypeStr=boolean  ZeroCross=off
  Subsystem : Subsystem
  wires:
  Constant1/1 -> Relational Operator/2
  Constant/1 -> Relational Operator/1
  Relational Operator/1 -> Subsystem/Enable
  Var/1 -> Subsystem/1(In1)

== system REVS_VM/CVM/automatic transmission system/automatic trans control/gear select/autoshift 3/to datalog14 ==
  Var : Inport
  Constant : Constant  Value=VerboseSignal
  Constant1 : Constant  Value=VerboseLevel
  Relational Operator : RelationalOperator  OutDataTypeStr=boolean  ZeroCross=off
  Subsystem : Subsystem
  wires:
  Constant1/1 -> Relational Operator/2
  Constant/1 -> Relational Operator/1
  Relational Operator/1 -> Subsystem/Enable
  Var/1 -> Subsystem/1(In1)

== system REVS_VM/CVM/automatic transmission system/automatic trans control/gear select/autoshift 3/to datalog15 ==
  Var : Inport
  Constant : Constant  Value=VerboseSignal
  Constant1 : Constant  Value=VerboseLevel
  Relational Operator : RelationalOperator  OutDataTypeStr=boolean  ZeroCross=off
  Subsystem : Subsystem
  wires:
  Constant1/1 -> Relational Operator/2
  Constant/1 -> Relational Operator/1
  Relational Operator/1 -> Subsystem/Enable
  Var/1 -> Subsystem/1(In1)

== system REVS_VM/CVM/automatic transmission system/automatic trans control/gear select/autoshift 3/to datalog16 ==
  Var : Inport
  Constant : Constant  Value=VerboseSignal
  Constant1 : Constant  Value=VerboseLevel
  Relational Operator : RelationalOperator  OutDataTypeStr=boolean  ZeroCross=off
  Subsystem : Subsystem
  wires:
  Constant1/1 -> Relational Operator/2
  Constant/1 -> Relational Operator/1
  Relational Operator/1 -> Subsystem/Enable
  Var/1 -> Subsystem/1(In1)

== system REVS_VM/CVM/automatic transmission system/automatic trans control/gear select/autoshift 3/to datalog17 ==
  Var : Inport
  Constant : Constant  Value=VerboseSignal
  Constant1 : Constant  Value=VerboseLevel
  Relational Operator : RelationalOperator  OutDataTypeStr=boolean  ZeroCross=off
  Subsystem : Subsystem
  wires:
  Constant1/1 -> Relational Operator/2
  Constant/1 -> Relational Operator/1
  Relational Operator/1 -> Subsystem/Enable
  Var/1 -> Subsystem/1(In1)

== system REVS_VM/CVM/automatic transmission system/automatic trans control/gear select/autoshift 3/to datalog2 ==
  Var : Inport
  Constant : Constant  Value=VerboseSignal
  Constant1 : Constant  Value=VerboseLevel
  Relational Operator : RelationalOperator  OutDataTypeStr=boolean  ZeroCross=off
  Subsystem : Subsystem
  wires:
  Constant1/1 -> Relational Operator/2
  Constant/1 -> Relational Operator/1
  Relational Operator/1 -> Subsystem/Enable
  Var/1 -> Subsystem/1(In1)

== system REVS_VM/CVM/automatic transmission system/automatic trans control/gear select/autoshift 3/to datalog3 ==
  Var : Inport
  Constant : Constant  Value=VerboseSignal
  Constant1 : Constant  Value=VerboseLevel
  Relational Operator : RelationalOperator  OutDataTypeStr=boolean  ZeroCross=off
  Subsystem : Subsystem
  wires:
  Constant1/1 -> Relational Operator/2
  Constant/1 -> Relational Operator/1
  Relational Operator/1 -> Subsystem/Enable
  Var/1 -> Subsystem/1(In1)

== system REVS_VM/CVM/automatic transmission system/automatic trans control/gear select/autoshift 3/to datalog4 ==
  Var : Inport
  Constant : Constant  Value=VerboseSignal
  Constant1 : Constant  Value=VerboseLevel
  Relational Operator : RelationalOperator  OutDataTypeStr=boolean  ZeroCross=off
  Subsystem : Subsystem
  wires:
  Constant1/1 -> Relational Operator/2
  Constant/1 -> Relational Operator/1
  Relational Operator/1 -> Subsystem/Enable
  Var/1 -> Subsystem/1(In1)

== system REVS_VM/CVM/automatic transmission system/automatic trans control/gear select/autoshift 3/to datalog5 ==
  Var : Inport
  Constant : Constant  Value=VerboseSignal
  Constant1 : Constant  Value=VerboseLevel
  Relational Operator : RelationalOperator  OutDataTypeStr=boolean  ZeroCross=off
  Subsystem : Subsystem
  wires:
  Constant1/1 -> Relational Operator/2
  Constant/1 -> Relational Operator/1
  Relational Operator/1 -> Subsystem/Enable
  Var/1 -> Subsystem/1(In1)

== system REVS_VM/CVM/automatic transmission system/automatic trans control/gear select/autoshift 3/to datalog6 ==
  Var : Inport
  Constant : Constant  Value=VerboseSignal
  Constant1 : Constant  Value=VerboseLevel
  Relational Operator : RelationalOperator  OutDataTypeStr=boolean  ZeroCross=off
  Subsystem : Subsystem
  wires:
  Constant1/1 -> Relational Operator/2
  Constant/1 -> Relational Operator/1
  Relational Operator/1 -> Subsystem/Enable
  Var/1 -> Subsystem/1(In1)

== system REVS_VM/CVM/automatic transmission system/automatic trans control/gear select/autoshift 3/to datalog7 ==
  Var : Inport
  Constant : Constant  Value=VerboseSignal
  Constant1 : Constant  Value=VerboseLevel
  Relational Operator : RelationalOperator  OutDataTypeStr=boolean  ZeroCross=off
  Subsystem : Subsystem
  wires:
  Constant1/1 -> Relational Operator/2
  Constant/1 -> Relational Operator/1
  Relational Operator/1 -> Subsystem/Enable
  Var/1 -> Subsystem/1(In1)

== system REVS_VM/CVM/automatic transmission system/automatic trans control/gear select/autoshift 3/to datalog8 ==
  Var : Inport
  Constant : Constant  Value=VerboseSignal
  Constant1 : Constant  Value=VerboseLevel
  Relational Operator : RelationalOperator  OutDataTypeStr=boolean  ZeroCross=off
  Subsystem : Subsystem
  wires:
  Constant1/1 -> Relational Operator/2
  Constant/1 -> Relational Operator/1
  Relational Operator/1 -> Subsystem/Enable
  Var/1 -> Subsystem/1(In1)

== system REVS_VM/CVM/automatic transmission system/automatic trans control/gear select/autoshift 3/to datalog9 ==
  Var : Inport
  Constant : Constant  Value=VerboseSignal
  Constant1 : Constant  Value=VerboseLevel
  Relational Operator : RelationalOperator  OutDataTypeStr=boolean  ZeroCross=off
  Subsystem : Subsystem
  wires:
  Constant1/1 -> Relational Operator/2
  Constant/1 -> Relational Operator/1
  Relational Operator/1 -> Subsystem/Enable
  Var/1 -> Subsystem/1(In1)
